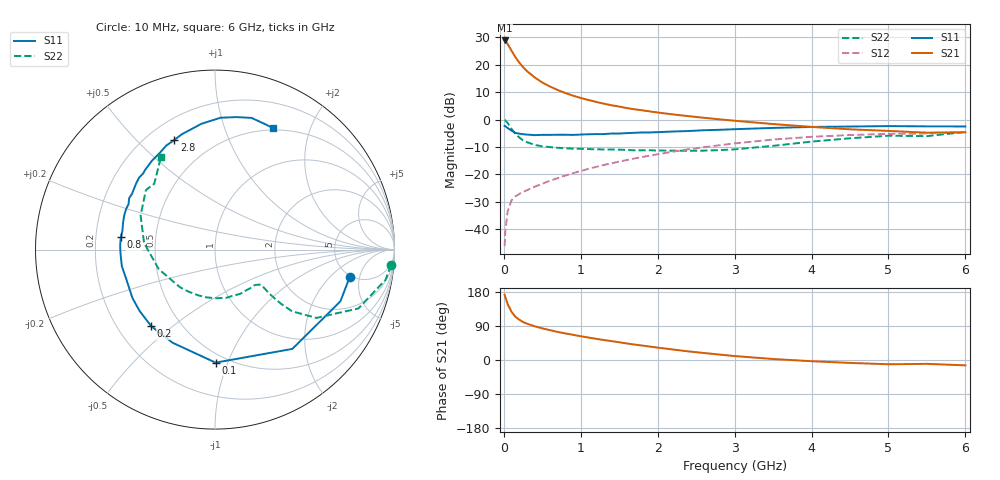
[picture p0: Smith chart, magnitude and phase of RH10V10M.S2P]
! SIEMENS Small Signal Semiconductors
! BFR106
! Si NPN RF Bipolar Junction Transistor in SOT23
! VCE = 10 V  IC = 10 mA
! Common Emitter S-Parameters:  August  1996
# GHz  S  MA  R  50
!  f  S11  S21  S12  S22
! GHz  MAG  ANG  MAG  ANG  MAG  ANG  MAG  ANG
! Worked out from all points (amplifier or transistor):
!   36 points, 10 MHz to 6 GHz, reference 50 ohm
!   highest |S21| = 28.9 dB at 10 MHz (marker M1)
!   |S21| within 3 dB of that: start of sweep to 84.69 MHz
!   unconditionally stable (mu >= 1): 503.3 MHz to 1.985 GHz; 5.355 GHz to end of sweep
!   at 250 MHz: K = 0.70, MSG = 22.8 dB, |S12| = -26.4 dB
!   at 1.4 GHz: K = 1.08, MAG = 8.8 dB, |S12| = -15.9 dB
!   at 6 GHz: K = 1.00, MAG = -0.5 dB, |S12| = -4.5 dB
!   S11 on the Smith chart (normalised r, x): 10 MHz: 4.86, -3.57; 100 MHz: 0.43, -0.91; 200 MHz: 0.34, -0.42; 800 MHz: 0.31, +0.06; 2.8 GHz: 0.31, +0.65; 6 GHz: 0.48, +1.48
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0.01  0.7663 -11.4  27.85 172.1  0.0049 86.1  0.9844 -5.0
0.02  0.7559 -22.4  27.24 165.8  0.0095 79.1  0.9653 -10.0
0.05  0.7012 -52.1  23.9 147.3  0.0212 66.9  0.8637 -22.3
0.1  0.6298 -89.7  18.11 127.3  0.0337 54.2  0.681 -34.0
0.15  0.5702 -114.4  13.8 114.1  0.0398 48.7  0.5496 -38.7
0.2  0.5553 -129.8  11.04 106.4  0.044 48.1  0.4728 -39.4
0.25  0.5414 -141.1  9.06 100.2  0.0479 47.8  0.4192 -39.2
0.3  0.5331 -149.7  7.689 96.0  0.0514 49.6  0.3874 -39.0
0.4  0.521 -161.5  5.912 89.2  0.0595 52.8  0.3465 -37.9
0.5  0.5271 -169.9  4.755 83.5  0.0676 55.8  0.3253 -37.4
0.6  0.5268 -177.1  4.014 78.6  0.0766 58.2  0.315 -38.2
0.8  0.5292 172.5  3.054 70.2  0.0954 61.2  0.2992 -41.2
0.9  0.5264 168.3  2.734 66.4  0.1053 62.2  0.2948 -42.9
1.1  0.5405 159.4  2.28 59.2  0.1265 63.6  0.29 -48.5
1.3  0.5443 152.2  1.954 52.7  0.1487 63.8  0.2853 -54.1
1.6  0.5667 142.3  1.624 43.6  0.183 63.0  0.2793 -64.5
2.2  0.6068 125.5  1.244 27.7  0.2602 58.2  0.2712 -89.8
2.8  0.6513 110.4  1.014 14.4  0.3404 50.5  0.2772 -122.5
3.5  0.7052 96.1  0.83 2.6  0.4327 39.5  0.3319 -160.9
4.5  0.7479 80.8  0.665 -7.7  0.5225 21.8  0.4563 155.3
5.5  0.7528 68.5  0.578 -10.2  0.5574 9.4  0.4991 132.7
6  0.7502 64.5  0.587 -14.1  0.5965 1.4  0.597 120.3
